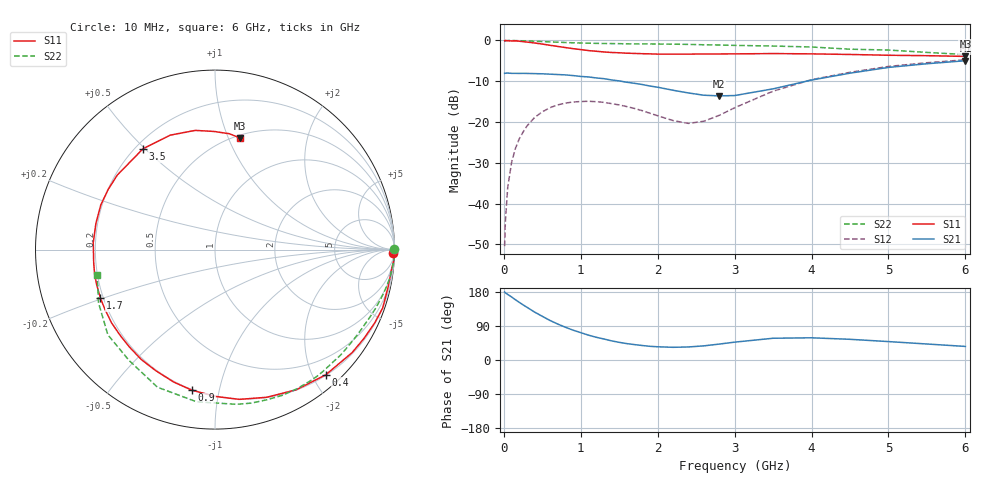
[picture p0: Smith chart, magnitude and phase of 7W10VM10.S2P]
! Infineon Technologies  Discrete & RF Semiconductors
! BFS17W
! Si NPN RF Bipolar Junction Transistor in SOT323
! VCE = 10 V  IC = 0.1 mA
! Common Emitter S-Parameters:  August  1999
# GHz  S  MA  R  50
!  f  S11  S21  S12  S22
! GHz  MAG  ANG  MAG  ANG  MAG  ANG  MAG  ANG
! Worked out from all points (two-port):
!   36 points, 10 MHz to 6 GHz, reference 50 ohm
!   highest |S21| = -4.97 dB at 6 GHz (marker M1); lowest = -13.6 dB at 2.8 GHz (marker M2)
!   |S21| within 3 dB of the highest: 4.518 GHz to end of sweep
!   lowest |S11| = -3.9 dB at 6 GHz (marker M3), VSWR 4.52, Z = 26.4 + j55.3 ohm
!   |S11| at or under -10 dB: nowhere
!   |S22| runs from -3.5 to 0.0 dB; largest |S21 - S12| = 0.4
!   S11 on the Smith chart (normalised r, x): 10 MHz: 31, -94; 400 MHz: 0.21, -2.20; 900 MHz: 0.20, -0.83; 1.7 GHz: 0.19, -0.20; 3.5 GHz: 0.23, +0.49; 6 GHz: 0.53, +1.11
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0.01  0.9937 -1.1  0.395 179.4  0.003 86.1  0.9999 0.2
0.02  0.9999 -2.8  0.397 177.3  0.006 92.9  0.9857 -0.5
0.05  0.9904 -6.2  0.398 173.1  0.0156 86.7  0.9991 -1.5
0.1  0.9867 -12.2  0.395 166.5  0.0317 82.3  0.9992 -3.2
0.15  0.9894 -19.2  0.395 159.1  0.0472 78.0  0.9951 -4.7
0.2  0.9789 -24.7  0.394 152.2  0.0621 74.4  0.9926 -6.3
0.3  0.9556 -36.9  0.394 139.2  0.0893 66.7  0.9862 -9.3
0.4  0.9313 -48.5  0.392 126.4  0.1137 59.7  0.9778 -12.2
0.6  0.8721 -70.6  0.386 104.3  0.1498 47.1  0.9601 -17.6
0.9  0.7935 -99.4  0.371 78.7  0.1759 31.9  0.9362 -25.3
1.1  0.7511 -116.0  0.357 65.6  0.1796 24.3  0.9255 -30.3
1.4  0.7122 -138.0  0.328 50.5  0.168 16.0  0.9154 -37.7
1.7  0.6932 -157.0  0.298 40.6  0.1464 12.5  0.907 -45.7
2.2  0.6794 176.6  0.245 33.5  0.1041 24.2  0.9001 -59.3
2.4  0.6794 167.5  0.227 34.4  0.0961 38.1  0.8946 -65.1
2.8  0.683 150.5  0.209 42.0  0.1207 65.6  0.8789 -76.7
3.5  0.6904 125.5  0.255 57.4  0.2388 75.5  0.8542 -96.9
4  0.6846 111.3  0.327 58.6  0.3304 69.4  0.831 -112.7
4.5  0.6732 99.4  0.397 54.6  0.4068 61.2  0.7813 -127.8
5  0.6584 90.5  0.467 48.6  0.4799 53.1  0.7627 -141.5
5.5  0.6504 83.0  0.518 42.2  0.5331 45.1  0.7134 -155.5
6  0.6374 77.2  0.564 35.8  0.5795 37.9  0.6713 -167.7
